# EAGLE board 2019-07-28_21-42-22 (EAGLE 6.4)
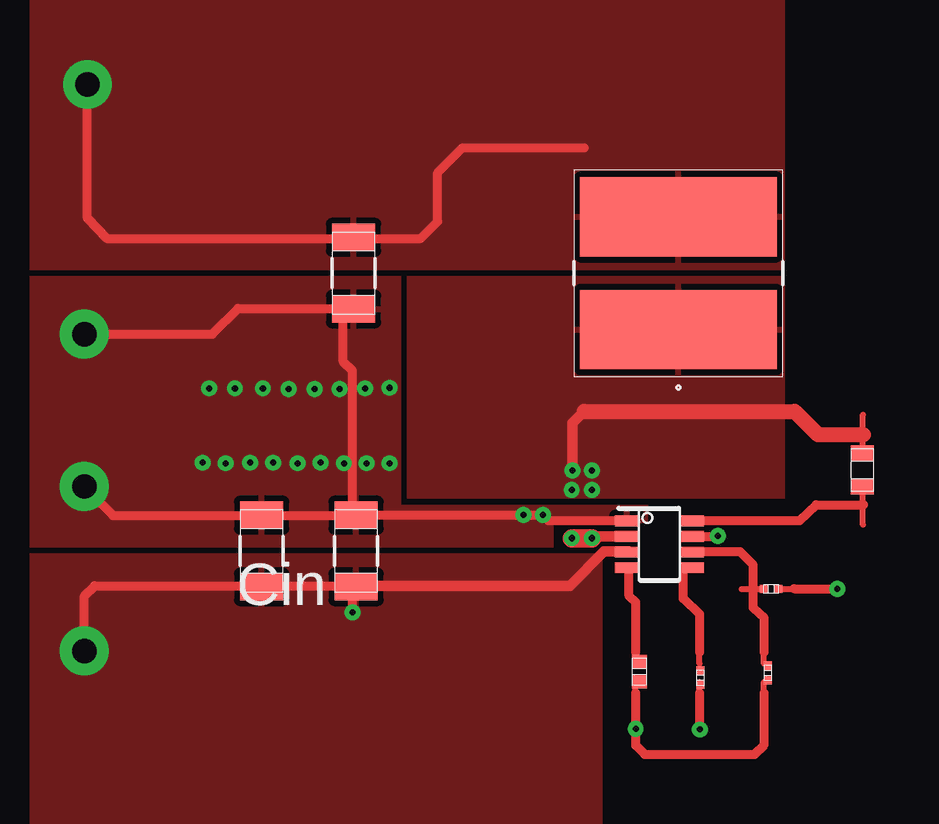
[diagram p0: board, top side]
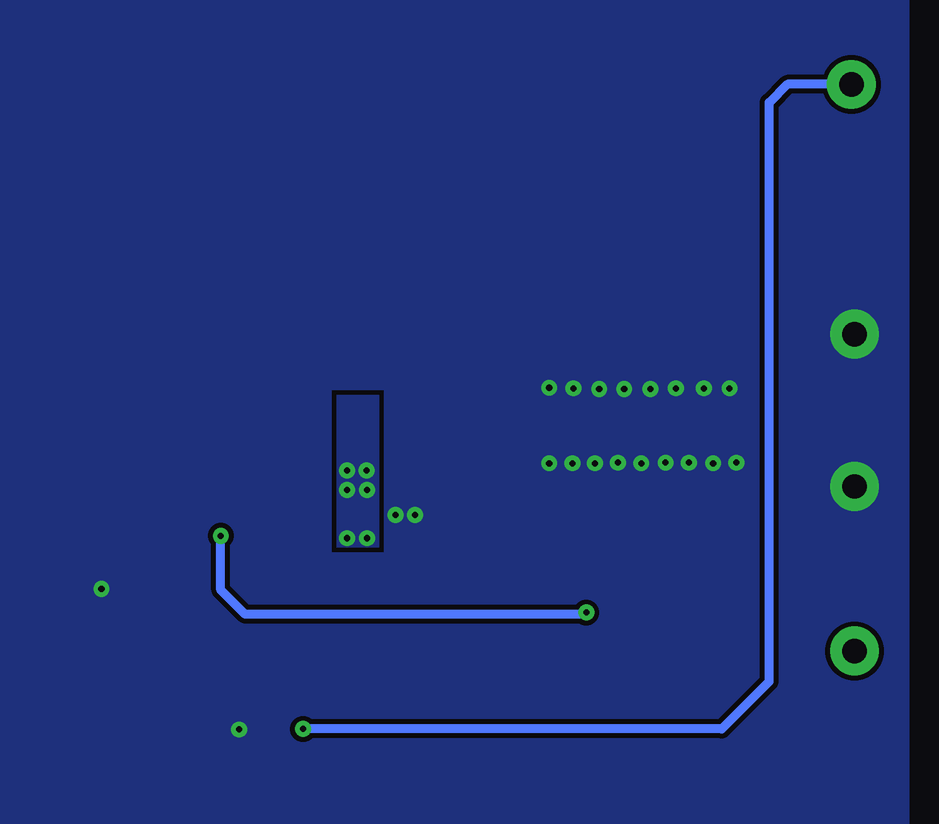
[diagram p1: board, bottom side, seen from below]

No outline drawn. Coordinates in mm, seen from the top.
Copper layers ((1*2)+(15*16)): TOP / INTERNAL1 / layer 15 / BOTTOM

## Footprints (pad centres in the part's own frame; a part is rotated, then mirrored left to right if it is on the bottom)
0603 = smd 0.66 x 0.965: 1 -0.699,0; 2 0.699,0
1206_190 = smd 1.118 x 1.803: 1 -1.499,0; 2 1.499,0
1206 = smd 1.118 x 1.803: 1 -1.499,0; 2 1.499,0
0201 = smd 0.356 x 0.33: 1 -0.292,0; 2 0.292,0
TP-1502 = drill 0.813 round: 1 0,0
VLP8040 = smd 3.302 x 8.204: 1 -2.349,0; 2 2.349,0
0402 = smd 0.559 x 0.61: 1 -0.419,0; 2 0.419,0
DDF0008A_N = smd 1 x 0.45: 1 -1.35,0.975; 2 -1.35,0.325; 3 -1.35,-0.325; 4 -1.35,-0.975; 5 1.35,-0.975; 6 1.35,-0.325; 7 1.35,0.325; 8 1.35,0.975

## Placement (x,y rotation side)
Cbst  [0603]  60.88,50.72 270 top
Cin_1  [1206_190]  39.78,47.35 90 top
Cin_2  [1206_190]  35.84,47.35 90 top
Cout  [1206]  39.67,58.93 270 top
Css  [0201]  54.13,42.06 270 top
GND  [TP-1502]  28.45,50.01 90 top
GND1  [TP-1502]  28.45,56.36 90 top
L1  [VLP8040]  53.21,58.93 90 top
Rfbb  [0201]  57.07,45.77 0 top
Rfbt  [0201]  56.95,42.27 90 top
Rpg  [0402]  51.59,42.32 90 top
U1  [DDF0008A_N]  52.43,47.62 0 top
VIN  [TP-1502]  28.45,43.13 90 top
VOUT  [TP-1502]  28.57,66.78 90 top

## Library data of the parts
Cbst = ultra-librarian; RefDes: Cbst; Type: C0603C104Z3VACTU
Cin_1 Cin_2 = ultra-librarian
Cout = ultra-librarian; RefDes: Cout; Type: C3216X5R1E476M160AC
Css = ultra-librarian; RefDes: Css; Type: GRM033R71A822KA01D
GND = ultra-librarian; RefDes: GND; Type: TP-1502
GND1 = ultra-librarian; RefDes: GND1; Type: TP-1502
L1 = ultra-librarian; RefDes: L1; Type: VLP8040T-3R3N
Rfbb = ultra-librarian; RefDes: Rfbb; Type: RC0201FR-0710KL
Rfbt = ultra-librarian; RefDes: Rfbt; Type: RC0201FR-0756K2L
Rpg = ultra-librarian; RefDes: Rpg; Type: CRCW0402100KFKED
U1 = ultra-librarian; RefDes: U1; Type: TPS563210ADDFR
VIN = ultra-librarian; RefDes: VIN; Type: TP-1502
VOUT = ultra-librarian; RefDes: VOUT; Type: TP-1502

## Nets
0: Cin_1.2 Cin_2.2 Cout.2 Css.2 GND1.1 GND.1 Rfbb.2 U1.1
2: Rfbb.1 Rfbt.2 U1.6
3: Cin_1.1 Cin_2.1 U1.3 U1.7 VIN.1
4: Cout.1 L1.2 Rfbt.1 Rpg.1 VOUT.1
5: Cbst.1 L1.1 U1.2
7: Cbst.2 U1.8
9: Rpg.2 U1.4
11: Css.1 U1.5

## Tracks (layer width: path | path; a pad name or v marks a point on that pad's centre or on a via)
0  (via drill 0.25 pad 0.61, 1.02 pad 2.03)
  TOP 0.254: 57.56,45.76 58.5,45.76 | 54.09,40.95 54.09,41.88
  TOP 0.381: 39.62,48.82 39.62,54.86 39.24,55.24 39.24,57.45 34.85,57.45 33.78,56.39 v28.45,56.39 | 39.62,48.82 39.62,48.84 v46.76,48.84 v47.57,48.84 47.78,48.62 51.16,48.62 | v28.45,50.04 29.64,48.82 39.62,48.82 | 58.04,45.77 v59.84,45.77 | v54.1,39.9 54.1,41.43
  other vias: 33.66,54.13 34.72,54.13 35.89,54.13 36.96,54.1 38.05,54.1 39.09,54.1 40.16,54.13 41.17,54.15 33.38,51.03 34.34,51 35.36,51.03 36.32,51.03 37.34,51 38.3,51.03 39.27,51 40.21,51 41.17,51
  pour TOP (rank 6): 26.16,58.8 41.66,58.8 41.66,49.28 51.94,49.28 51.94,48.51 48.01,48.51 48.01,47.5 26.16,47.5
  pour BOTTOM (rank 5): 26.16,85.6 26.16,26.16 75.44,26.16 75.44,85.6
2
  TOP 0.254: 55.85,45.76 56.79,45.76 | 56.78,42.65 56.78,43.59
  TOP 0.381: 53.42,47.32 55.78,47.32 56.34,46.76 56.34,45.77 56.34,44.98 56.79,44.55 56.79,43.13
3  (via drill 0.25 pad 0.61, 1.02 pad 2.03)
  TOP 0.381: v39.62,44.78 39.62,45.9 28.88,45.9 28.45,45.47 v28.45,43.18 | v54.86,47.98 54.84,47.95 53.42,47.95
  TOP 0.432: 39.62,45.9 48.69,45.9 50.11,47.32 51.16,47.32
  BOTTOM 0.381: v54.86,47.98 54.86,45.72 53.85,44.7 39.7,44.7
  pour TOP (rank 2): 50.04,47.24 50.04,30.48 26.16,30.48 26.16,47.24
4  (via drill 0.25 pad 0.61, 1.02 pad 2.03)
  TOP 0.254: 56.78,40.95 56.78,41.88 | 51.42,40.95 51.42,41.88
  TOP 0.381: 56.79,41.43 56.79,39.27 56.39,38.86 51.82,38.86 51.44,39.24 v51.44,39.93 51.44,41.43 | 49.28,64.16 44.22,64.16 43.18,63.12 43.18,61.09 42.47,60.38 39.24,60.38 29.39,60.38 28.57,61.21 v28.57,66.8
  BOTTOM 0.381: v51.44,39.93 33.98,39.93 32,41.91 32,66.04 31.24,66.8 v28.57,66.8
  pour TOP (rank 4): 26.16,59.05 57.66,59.05 57.66,73.66 26.16,73.66
5  (via drill 0.25 pad 0.61)
  TOP 0.254: 60.91,51.33 60.91,53.03
  TOP 0.432: 49.28,53.16 48.79,52.68 v48.79,50.7 | v49.61,47.88 49.68,47.95 51.16,47.95
  TOP 0.635: 49.28,53.16 58.06,53.16 59.03,52.2 60.94,52.2
  TOP 0.762: v48.77,47.88 v49.61,47.88
  other vias: 48.77,49.89 49.61,49.89 49.61,50.7
  pour TOP (rank 3): 57.66,58.8 41.91,58.8 41.91,49.53 57.66,49.53
  pour BOTTOM: 48.26,47.5 48.26,53.85 50.04,53.85 50.04,47.5
7
  TOP 0.254: 60.91,48.44 60.91,50.14
  TOP 0.381: 53.42,48.62 58.27,48.62 58.95,49.28 60.94,49.28
9
  TOP 0.254: 51.42,42.65 51.42,43.59
  TOP 0.381: 51.16,46.66 51.16,45.47 51.44,45.21 51.44,43.13
11
  TOP 0.254: 54.09,42.65 54.09,43.59
  TOP 0.381: 54.1,43.13 54.1,44.7 53.42,45.36 53.42,46.66

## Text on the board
ASSYNOTES: Note: | Min. Clearance: 10 mil | Min. | Track Width : 10 mil | Cin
